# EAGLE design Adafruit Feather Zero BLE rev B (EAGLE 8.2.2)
COMPANY: ADAFRUIT INDUSTRIES; DRAWN: KTOWN; REV: B
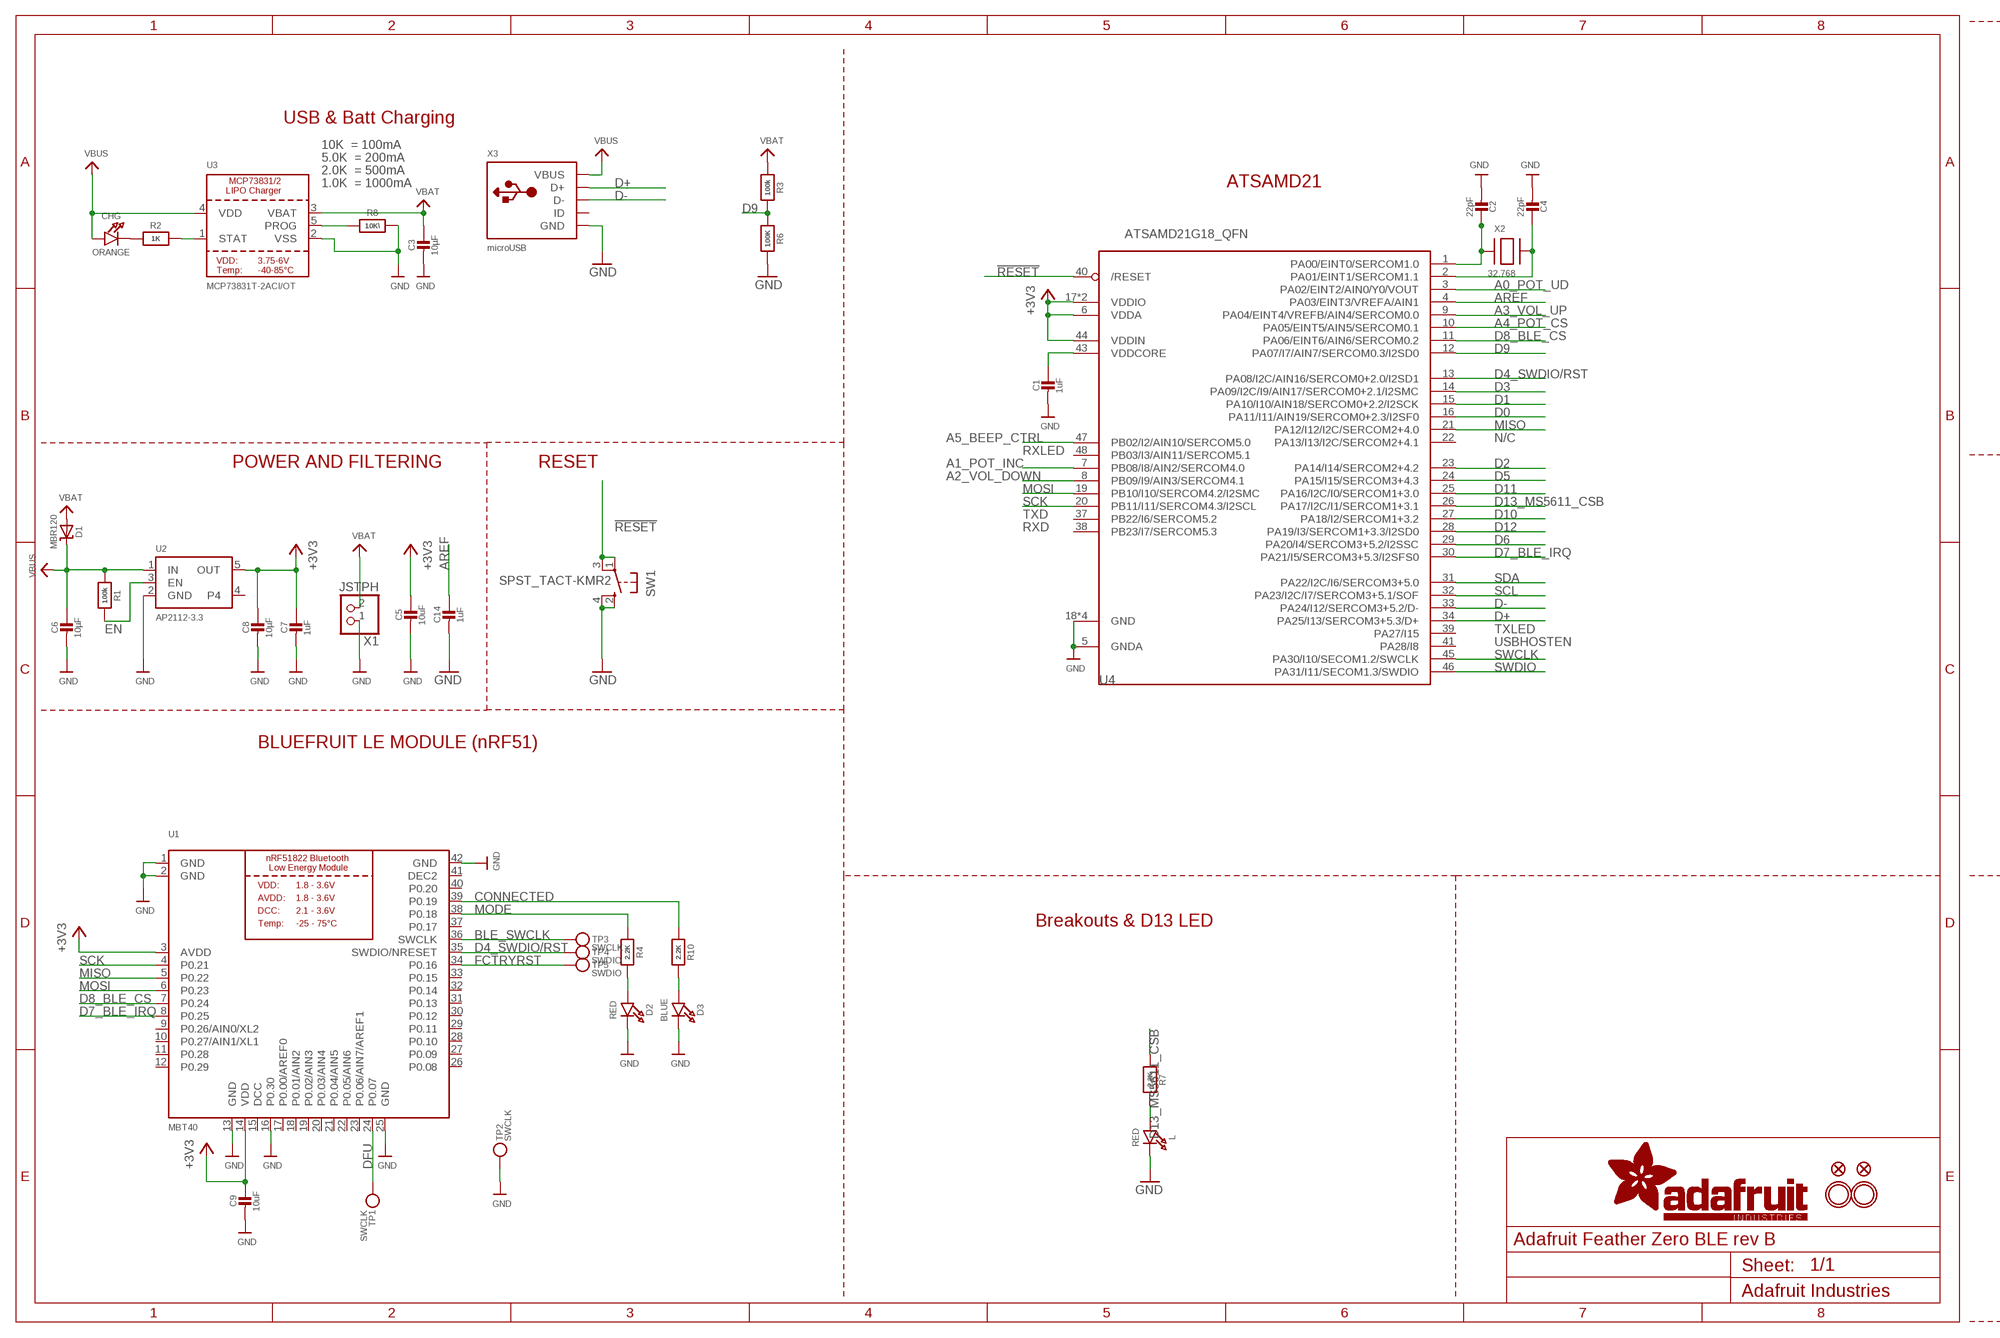
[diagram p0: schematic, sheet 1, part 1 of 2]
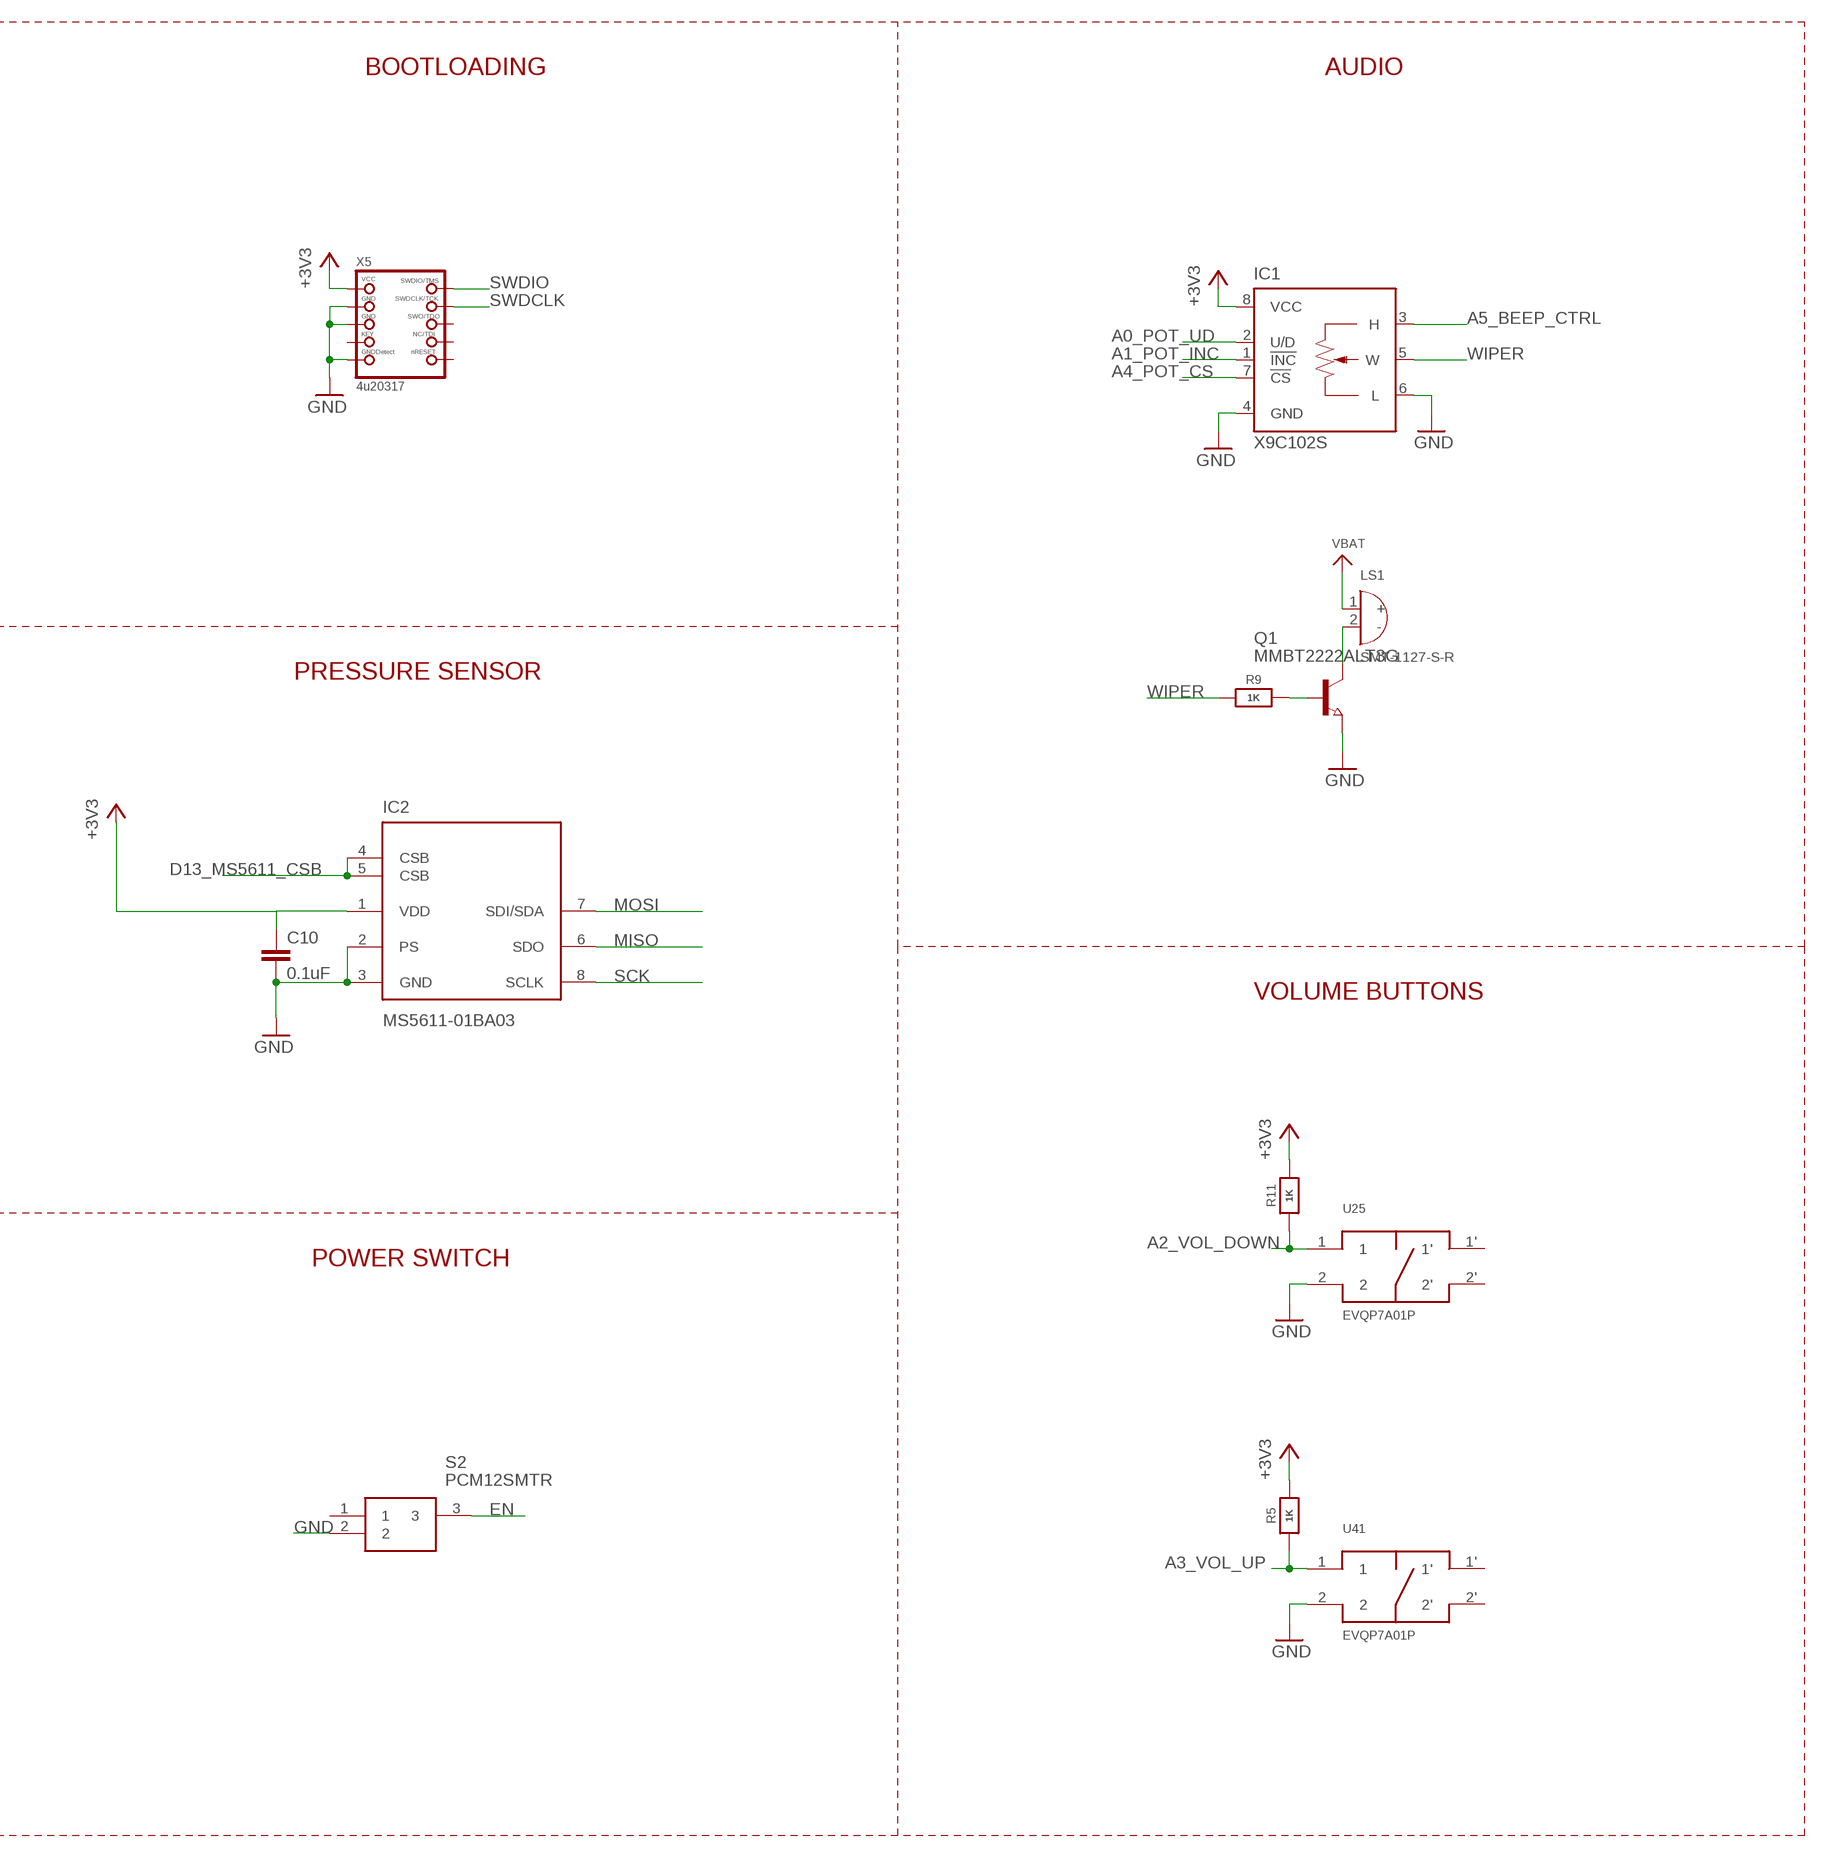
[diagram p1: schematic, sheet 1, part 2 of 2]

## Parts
C1  1uF  CAP_CERAMIC0603_NO  [0603-NO]
C2  22pF  CAP_CERAMIC0603_NO  [0603-NO]
C3  10µF  CAP_CERAMIC0805-NOOUTLINE  [0805-NO]
C4  22pF  CAP_CERAMIC0603_NO  [0603-NO]
C5  10uF  CAP_CERAMIC0805-NOOUTLINE  [0805-NO]
C6  10µF  CAP_CERAMIC0805-NOOUTLINE  [0805-NO]
C7  1uF  CAP_CERAMIC0603_NO  [0603-NO]
C8  10µF  CAP_CERAMIC0805-NOOUTLINE  [0805-NO]
C9  10uF  CAP_CERAMIC0805-NOOUTLINE  [0805-NO]
C10  0.1uF  C-EUC0805K  [C0805K]
C14  1uF  CAP_CERAMIC0603_NO  [0603-NO]
CHG  ORANGE  LED0805_NOOUTLINE  [CHIPLED_0805_NOOUTLINE]
D1  MBR120  DIODE-SCHOTTKYSOD-123  [SOD-123]
D2  RED  LED0805_NOOUTLINE  [CHIPLED_0805_NOOUTLINE]
D3  BLUE  LED0805_NOOUTLINE  [CHIPLED_0805_NOOUTLINE]
IC1  X9C102S  [SOIC08]
IC2  MS5611-01BA03  MS5611-01BA03UNO  [SON125P300X500X100-8N]
L  RED  LED0805_NOOUTLINE  [CHIPLED_0805_NOOUTLINE]
LS1  SMT-1127-S-R  [XDCR_SMT-1127-S-R]
Q1  MMBT2222ALT3G  NPN-TRANSISTOR_SOT23  [SOT23]
R1  100k  RESISTOR_0603_NOOUT  [0603-NO]
R2  1K  RESISTOR_0603_NOOUT  [0603-NO]
R3  100k  RESISTOR_0603_NOOUT  [0603-NO]
R4  2.2K  RESISTOR_0603_NOOUT  [0603-NO]
R5  1K  RESISTOR_0603_NOOUT  [0603-NO]
R6  100K  RESISTOR_0603_NOOUT  [0603-NO]
R7  2.2K  RESISTOR_0603_NOOUT  [0603-NO]
R8  10K\  RESISTOR_0603_NOOUT  [0603-NO]
R9  1K  RESISTOR_0603_NOOUT  [0603-NO]
R10  2.2K  RESISTOR_0603_NOOUT  [0603-NO]
R11  1K  RESISTOR_0603_NOOUT  [0603-NO]
S2  PCM12SMTR  [PCM12SMTR_1]
SW1  SPST_TACT-KMR2  [KMR2]
TP1  SWCLK  TESTPOINT1.5X2.0MM_NOCREAM  [PAD-1.5X2.0]
TP2  SWCLK  TESTPOINT1.5X2.0MM_NOCREAM  [PAD-1.5X2.0]
TP3  SWCLK  TESTPOINT1.5X2.0MM_NOCREAM  [PAD-1.5X2.0]
TP4  SWDIO  TESTPOINT1.5X2.0MM_NOCREAM  [PAD-1.5X2.0]
TP5  SWDIO  TESTPOINT1.5X2.0MM_NOCREAM  [PAD-1.5X2.0]
U1  MBT40  NRF51822_MODULE_MDBT40  [BLE_MODULE_RAYTAC_MDBT40]
U2  AP2112-3.3  VREG_SOT23-5  [SOT23-5]
U3  MCP73831T-2ACI/OT  MCP73831/2  [SOT23-5]
U4  ATSAMD21G18_QFN  ATSAMD21J_QFN  [TQFN48_7MM]
U25  EVQP7A01P  [EVQP7A01P]
U41  EVQP7A01P  [EVQP7A01P]
U$31  MOUNTINGHOLE2.5  [MOUNTINGHOLE_2.5_PLATED]
U$32  MOUNTINGHOLE2.5  [MOUNTINGHOLE_2.5_PLATED]
U$34  FIDUCIAL""  [FIDUCIAL_1MM]
U$35  FIDUCIAL""  [FIDUCIAL_1MM]
X1  JSTPH  CON_JST_PH_2PIN  [JSTPH2]
X2  32.768  XTAL-3.2X1.5  [XTAL3215]
X3  microUSB  USB_MICRO_20329_V2  [4UCONN_20329_V2]
X5  4u20317  JTAG-CORTEXBOXPOSTS  [2X05_1.27MM_BOX_POSTS]

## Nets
!RESET: SW1.1(P) SW1.3(P1) U4.40(/RESET)
+3V3: C5.1 C7.1 C8.1 C9.1 C10.1 IC1.8(VCC) IC2.1(VDD) R5.2 R11.2 U1.3(AVDD) U1.14(VDD) U2.5(OUT) U4.6(VDDA) U4.17(VDDIO) U4.36(VDDIO) U4.44(VDDIN) X5.1(VCC)
A0_POT_UD: IC1.2(U/D) U4.3(PA02/EINT2/AIN0/Y0/VOUT)
A1_POT_INC: IC1.1(!INC) U4.7(PB08/I8/AIN2/SERCOM4.0)
A2_VOL_DOWN: R11.1 U4.8(PB09/I9/AIN3/SERCOM4.1) U25.1
A3_VOL_UP: R5.1 U4.9(PA04/EINT4/VREFB/AIN4/SERCOM0.0) U41.1
A4_POT_CS: IC1.7(!CS) U4.10(PA05/EINT5/AIN5/SERCOM0.1)
A5_BEEP_CTRL: IC1.3(H) U4.47(PB02/I2/AIN10/SERCOM5.0)
AREF: C14.1 U4.4(PA03/EINT3/VREFA/AIN1)
BLE_SWCLK: TP3.P$1 U1.36(SWCLK)
CONNECTED: R10.1 U1.39(P0.19)
D0: U4.16(PA11/I11/AIN19/SERCOM0+2.3/I2SF0)
D1: U4.15(PA10/I10/AIN18/SERCOM0+2.2/I2SCK)
D2: U4.23(PA14/I14/SERCOM2+4.2)
D3: U4.14(PA09/I2C/I9/AIN17/SERCOM0+2.1/I2SMC)
D4_SWDIO/RST: TP4.P$1 U1.35(SWDIO/NRESET) U4.13(PA08/I2C/AIN16/SERCOM0+2.0/I2SD1)
D5: U4.24(PA15/I15/SERCOM3+4.3)
D6: U4.29(PA20/I4/SERCOM3+5.2/I2SSC)
D7_BLE_IRQ: U1.8(P0.25) U4.30(PA21/I5/SERCOM3+5.3/I2SFS0)
D8_BLE_CS: U1.7(P0.24) U4.11(PA06/EINT6/AIN6/SERCOM0.2)
D9: R3.2 R6.1 U4.12(PA07/I7/AIN7/SERCOM0.3/I2SD0)
D10: U4.27(PA18/I2/SERCOM1+3.2)
D11: U4.25(PA16/I2C/I0/SERCOM1+3.0)
D12: U4.28(PA19/I3/SERCOM1+3.3/I2SD0)
D13_MS5611_CSB: IC2.4(CSB) IC2.5(CSB) R7.1 U4.26(PA17/I2C/I1/SERCOM1+3.1)
D+: U4.34(PA25/I13/SERCOM3+5.3/D+) X3.D+
D-: U4.33(PA24/I12/SERCOM3+5.2/D-) X3.D-
DFU: TP1.P$1 U1.24(P0.07)
EN: R1.2 S2.3 U2.3(EN)
FCTRYRST: TP5.P$1 U1.34(P0.16)
GND: C1.2 C2.2 C3.2 C4.2 C5.2 C6.2 C7.2 C8.2 C9.2 C10.2 C14.2 D2.C D3.C IC1.4(GND) IC1.6(L) IC2.2(PS) IC2.3(GND) L.C Q1.2(E) R6.2 R8.2 S2.2 SW1.2(S) SW1.4(S1) TP2.P$1 U1.1(GND) U1.2(GND) U1.13(GND) U1.16(P0.30) U1.25(GND) U1.42(GND) U2.2(GND) U3.2(VSS) U4.5(GNDA) U4.18(GND) U4.35(GND) U4.42(GND) U4.THERMAL(GND) U25.2 U41.2 X1.1 X3.BASE@1(GND) X3.BASE@2(GND) X3.GND X3.SPRT@1(GND) X3.SPRT@2(GND) X3.SPRT@3(GND) X3.SPRT@4(GND) X5.3(GND) X5.5(GND) X5.9(GNDDETECT)
MISO: IC2.6(SDO) U1.5(P0.22) U4.21(PA12/I12/I2C/SERCOM2+4.0)
MODE: R4.1 U1.38(P0.18)
MOSI: IC2.7(SDI/SDA) U1.6(P0.23) U4.19(PB10/I10/SERCOM4.2/I2SMC)
N$1: CHG.C R2.1
N$2: L.A R7.2
N$3: R2.2 U3.1(STAT)
N$4: R8.1 U3.5(PROG)
N$5: C2.1 U4.1(PA00/EINT0/SERCOM1.0) X2.P$1
N$6: D2.A R4.2
N$7: C4.1 U4.2(PA01/EINT1/SERCOM1.1) X2.P$2
N$8: D3.A R10.2
N$9: Q1.1(B) R9.2
N$10: LS1.2(-) Q1.3(C)
SCK: IC2.8(SCLK) U1.4(P0.21) U4.20(PB11/I11/SERCOM4.3/I2SCL)
SCL: U4.32(PA23/I2C/I7/SERCOM3+5.1/SOF)
SDA: U4.31(PA22/I2C/I6/SERCOM3+5.0)
SWCLK: U4.45(PA30/I10/SECOM1.2/SWCLK)
SWDCLK: X5.4(SWDCLK)
SWDIO: U4.46(PA31/I11/SECOM1.3/SWDIO) X5.2(SWDIO)
VBAT: C3.1 D1.A LS1.1(+) R3.1 U3.3(VBAT) X1.2
VBUS: C6.1 CHG.A D1.C R1.1 U2.1(IN) U3.4(VDD) X3.VBUS
VDDCORE: C1.1 U4.43(VDDCORE)
WIPER: IC1.5(W) R9.1
Unconnected: S2.1 U1.9(P0.26/AIN0/XL2) U1.10(P0.27/AIN1/XL1) U1.11(P0.28) U1.12(P0.29) U1.17(P0.00/AREF0) U1.18(P0.01/AIN2) U1.19(P0.02/AIN3) U1.20(P0.03/AIN4) U1.21(P0.04/AIN5) U1.22(P0.05/AIN6) U1.23(P0.06/AIN7/AREF1) U1.26(P0.08) U1.27(P0.09) U1.28(P0.10) U1.29(P0.11) U1.30(P0.12) U1.31(P0.13) U1.32(P0.14) U1.33(P0.15) U1.37(P0.17) U1.40(P0.20) U2.4 U4.22(PA13/I13/I2C/SERCOM2+4.1) U4.37(PB22/I6/SERCOM5.2) U4.38(PB23/I7/SERCOM5.3) U4.39(PA27/I15) U4.41(PA28/I8) U4.48(PB03/I3/AIN11/SERCOM5.1) U25.1' U25.2' U41.1' U41.2' X3.ID X5.6(SWO) X5.7(KEY) X5.8(TDI) X5.10(NRESET)

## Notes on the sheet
- BOOTLOADING | AUDIO
- USB & Batt Charging
- 10K  = 100mA
- 5.0K  = 200mA
- 2.0K  = 500mA
- 1.0K  = 1000mA | ATSAMD21
- N/C
- RXLED
- POWER AND FILTERING | RESET
- PRESSURE SENSOR
- TXD
- RXD
- TXLED
- USBHOSTEN
- VOLUME BUTTONS
- BLUEFRUIT LE MODULE (nRF51)
- POWER SWITCH
- Breakouts & D13 LED

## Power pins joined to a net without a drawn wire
DCC: U1.15(DCC)
DEC2: U1.41(DEC2)

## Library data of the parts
C1-C9 C14 = microbuilder:CAP_CERAMIC: Ceramic Capacitors
C10 = rcl:C-EU: CAPACITOR, European symbol
CHG D2 D3 L = microbuilder:LED: LED
D1 = microbuilder:DIODE-SCHOTTKY
IC1 = pot-xicor:X9C102*: Digital POTENTIOMETER; MF: INTERSIL; MPN: X9C102SIZ; OC_FARNELL: 1562072; OC_NEWARK: 79K8947
IC2 = Measurement-Specialties:MS5611-01BA03: Variometer Module, with stainless steel cap
LS1 = SMT-1127-S-R:SMT-1127-S-R: Audio Indicator Transducer Electromagnetic 3.6Vpk 100mA Solder Pad 2.5Vpk 2231Hz to 3231Hz Surface Mount; AVAILABILITY: Good; DESCRIPTION: Black Passive Electromagnetic SMD Buzzer 3V 80mA 2700Hz 92dB 9x3.2mm; MF: PUI Audio; MP: BOT-03D-BUJEON, SMT-1127-S-R; PACKAGE: None; PRICE: 1.43 USD
Q1 = semicon-smd-ipc:NPN-TRANSISTOR_: NPN TRANSISTOR
R1-R11 = microbuilder:RESISTOR: Resistors
S2 = PCM12SMTR:PCM12SMTR: C & K COMPONENTS - PCM12SMTR - SWITCH, SPDT, 0.3A, 6VDC, SMD Source: Datasheet; ALLIED_NUMBER: 70417448; ALLIED_PRICE/STOCK: http://www.alliedelec.com/c-k-components-pcm12smtr/70417448/; DESCRIPTION: C & K COMPONENTS - PCM12SMTR - SWITCH, SPDT, 0.3A, 6VDC, SMD; HEIGHT: mm; MANUFACTURER_NAME: C & K COMPONENTS; MANUFACTURER_PART_NUMBER: PCM12SMTR; RS_PART_NUMBER: 7931721P; RS_PRICE/STOCK: http://uk.rs-online.com/web/p/products/7931721P
SW1 = adafruit:SPST_TACT: SMT 6mm switch, EVQQ2 series http://www.ladyada.net/library/eagle
TP1-TP5 = microbuilder:TESTPOINT: Test Point
U1 = microbuilder:NRF51822_MODULE_MDBT40: nRF51822 Bluetooth Low Energy Module
U2 = microbuilder:VREG_SOT23-5: SOT23-5 Fixed Voltage Regulators Part Current Out V Out V In V Dropout θJA (°C/W) TJ (°C) Digikey Part No. ADP121 150mA 3.3V 3.4-5.5V 0.09V @ 150mA -- -- ADP121-AUJZ33R7CT-ND ADP121 150mA 3.0V 3.1-5.5V 0.09V @ 150mA -- -- ADP121-AUJZ30R7CT-ND ADP122 300mA 3.3V 3.4-5.5V 0.085V @ 300mA -- --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
U3 = microbuilder:MCP73831/2: MCP73831/2 LIPO Charger VDD: 3.75 - 6V Temp -40 - 85°C Programmable Charge Rate: 15-500mA NOTE: STAT is a tri-state logic output on the MCP73831 and an open-drain output on the MCP73832. SOT23-5 with 4.2V output and tri-state logic on STAT = MCP73831T-2ACI/OT
U4 = microbuilder:ATSAMD21J
U25 U41 = EVQP7A01P:EVQP7A01P: EVQP7A01P Tactile Switch Surface Mount Right Angle
U$31 U$32 = microbuilder:MOUNTINGHOLE: Mounting Hole; BOM: EXCLUDE
U$34 U$35 = microbuilder:FIDUCIAL: Fiducial Alignment Points; BOM: EXCLUDE
X1 = microbuilder:CON_JST_PH_2PIN: JST 2-Pin Right-Angle Connector
X2 = adafruit2:XTAL: Low cost SMT crystals, no capacitors included
X3 = microbuilder:USB: USB Connectors USBMINIB - Surface Mount Female Mini-B USB Connector 4UConnector: 06564
X5 = microbuilder:JTAG-CORTEX: Serial Wire (SW-DP) Connector Standard 0.05" 10-pin connector is for use with the Cortex M and Cortex A SWD (serial wire debugger) interface (SW-DP) Connectors 2x05_1.27MM_SMT - Inexpensive surface-mount header with bare pins, compatible with standard 10-pin SWD cables (4UCON: 16846)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

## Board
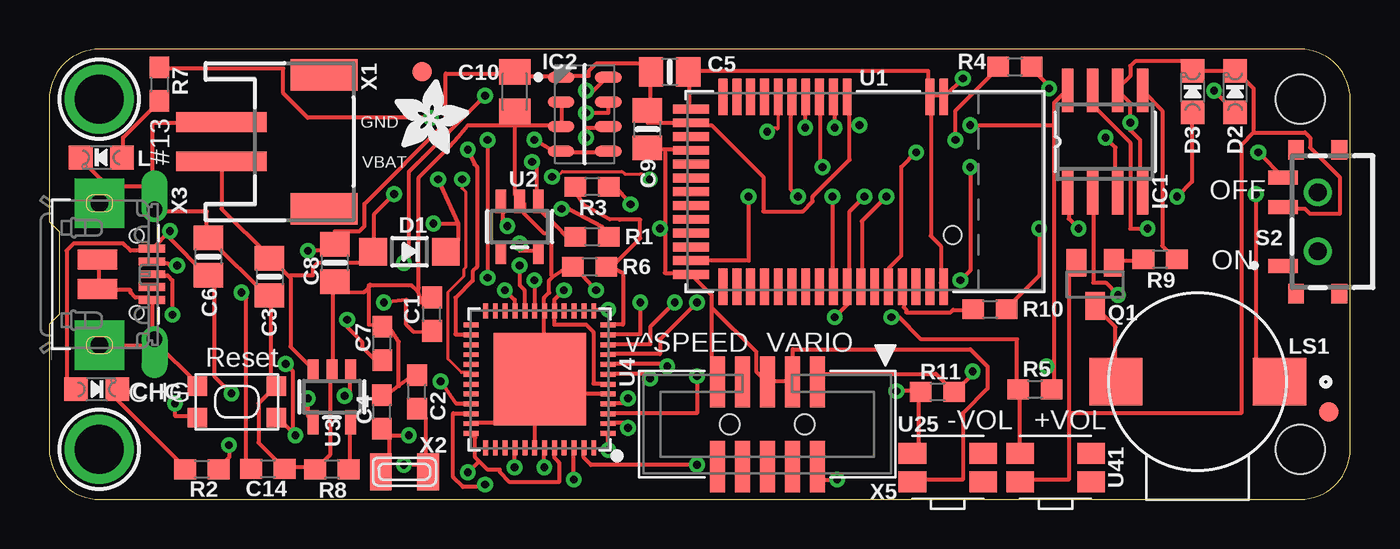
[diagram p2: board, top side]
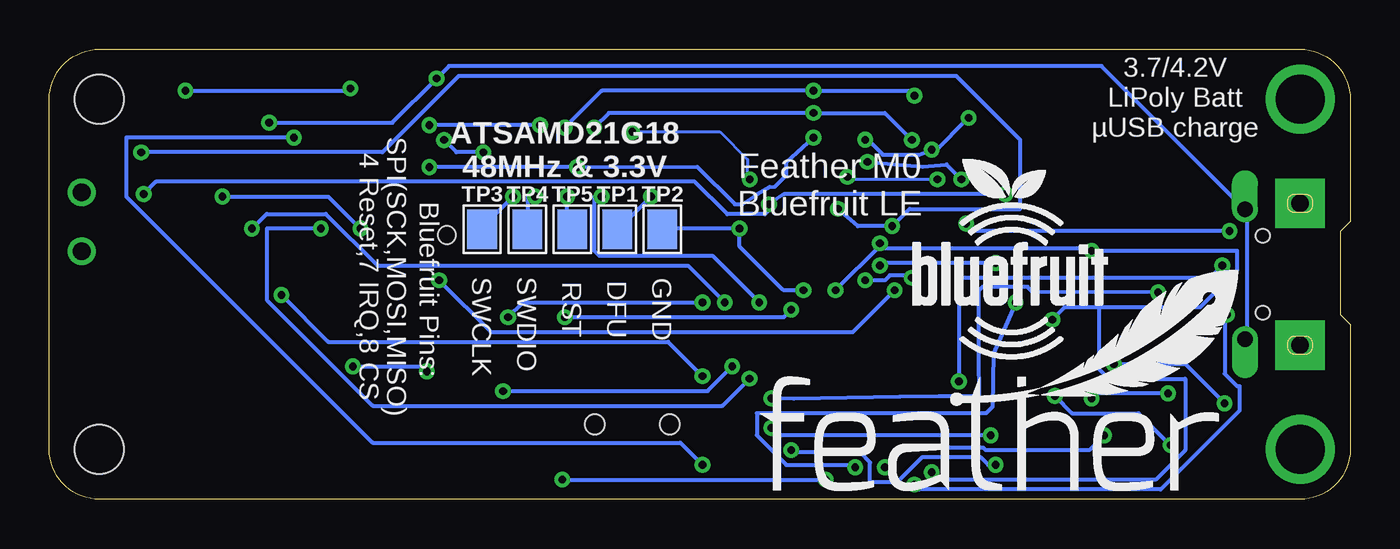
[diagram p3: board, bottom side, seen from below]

Size 66.04 x 22.86 mm. Coordinates in mm from the lower left corner, seen from the top.
Outline: 2.54,0 63.5,0 arc90 66.04,2.54 66.04,20.32 arc90 63.5,22.86 2.54,22.86 arc90 0,20.32 0,14.1 0.51,13.59 0.51,9.4 0,8.89 0,2.54 arc90 2.54,0
Copper layers (1*16): Top 0.035mm / dielectric 1.5mm / Bottom 0.035mm
Design rules "adafruit *": minimum track width 8mil, minimum drill 15.5mil, track to track 8mil, track to pad 8mil, pad to pad 8mil, via to via 8mil, smd to smd 8mil, copper to edge 10mil, drill to drill 8mil, minimum pad ring 10mil, minimum via ring 8mil, stop-mask expansion 2mil, vias tented up to drill 20mil, thermal gap 10mil
Holes 2.5 mm at 63.5,2.54 63.5,20.32

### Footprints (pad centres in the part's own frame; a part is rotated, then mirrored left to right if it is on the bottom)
0603-NO = smd 1.1 x 1: 1 -0.85,0; 2 0.85,0
0805-NO = smd 1.24 x 1.5: 1 -0.95,0; 2 0.95,0
C0805K = smd 1.3 x 1.6: 1 -1,0; 2 1,0
CHIPLED_0805_NOOUTLINE = smd 1.2 x 1.2: A 0,-1.05; C 0,1.05
SOD-123 = smd 1.4 x 1.4: A 1.85,0; C -1.85,0
SOIC08 = smd 0.6 x 2.2: 1 -1.905,-2.6; 2 -0.635,-2.6; 3 0.635,-2.6; 4 1.905,-2.6; 5 1.905,2.6; 6 0.635,2.6; 7 -0.635,2.6; 8 -1.905,2.6
SON125P300X500X100-8N = smd 1.35 x 0.55: 1 -1.2,1.875; 2 -1.2,0.625; 3 -1.2,-0.625; 4 -1.2,-1.875; 5 1.2,-1.875; 6 1.2,-0.625; 7 1.2,0.625; 8 1.2,1.875
XDCR_SMT-1127-S-R = smd 2.71 x 2.41: 1 -4.15,0; 2 4.15,0
SOT23 = smd 1 x 1.4: 1 -0.95,-1.1; 2 0.95,-1.1; 3 0,1.1
PCM12SMTR_1 = smd 0.7 x 1.5: 1 -2.25,1.75; 2 0.75,1.75; 3 2.25,1.75 | smd 1 x 0.8: 4 -3.65,1.1; 5 -3.65,-1.1; 6 3.65,1.1; 7 3.65,-1.1 | drill 0.9 pad 1.4: 8 -1.5,0; 9 1.5,0
KMR2 = smd 1 x 1: 1 2,0.8; 2 2,-0.8; 3 -2,0.8; 4 -2,-0.8
PAD-1.5X2.0 = smd 1.5 x 2: P$1 0,0
BLE_MODULE_RAYTAC_MDBT40 = smd 1.85 x 0.45: 1 -4.825,4; 2 -4.825,3.3; 3 -4.825,-0.9; 4 -4.825,-1.6; 5 -4.825,-2.3; 6 -4.825,-3; 7 -4.825,-3.7; 8 -4.825,-4.4; 9 -4.825,-5.1; 10 -4.825,-5.8; 11 -4.825,-6.5; 12 -4.825,-7.2; 26 4.825,-7.2; 27 4.825,-6.5; 28 4.825,-5.8; 29 4.825,-5.1; 30 4.825,-4.4; 31 4.825,-3.7; 32 4.825,-3; 33 4.825,-2.3; 34 4.825,-1.6; 35 4.825,-0.9; 36 4.825,-0.2; 37 4.825,0.5; 38 4.825,1.2; 39 4.825,1.9; 40 4.825,2.6; 41 4.825,3.3; 42 4.825,4 | smd 0.45 x 1.85: 13 -4.2,-8.825; 14 -3.5,-8.825; 15 -2.8,-8.825; 16 -2.1,-8.825; 17 -1.4,-8.825; 18 -0.7,-8.825; 19 0,-8.825; 20 0.7,-8.825; 21 1.4,-8.825; 22 2.1,-8.825; 23 2.8,-8.825; 24 3.5,-8.825; 25 4.2,-8.825 | hole 0.9: 2.2,4.45
SOT23-5 = smd 0.55 x 1.2: 1 -0.95,-1.3; 2 0,-1.3; 3 0.95,-1.3; 4 0.95,1.3; 5 -0.95,1.3
TQFN48_7MM = smd 0.25 x 0.75: 1 -2.75,-3.475; 2 -2.25,-3.475; 3 -1.75,-3.475; 4 -1.25,-3.475; 5 -0.75,-3.475; 6 -0.25,-3.475; 7 0.25,-3.475; 8 0.75,-3.475; 9 1.25,-3.475; 10 1.75,-3.475; 11 2.25,-3.475; 12 2.75,-3.475; 25 2.75,3.475; 26 2.25,3.475; 27 1.75,3.475; 28 1.25,3.475; 29 0.75,3.475; 30 0.25,3.475; 31 -0.25,3.475; 32 -0.75,3.475; 33 -1.25,3.475; 34 -1.75,3.475; 35 -2.25,3.475; 36 -2.75,3.475 | smd 0.75 x 0.25: 13 3.475,-2.75; 14 3.475,-2.25; 15 3.475,-1.75; 16 3.475,-1.25; 17 3.475,-0.75; 18 3.475,-0.25; 19 3.475,0.25; 20 3.475,0.75; 21 3.475,1.25; 22 3.475,1.75; 23 3.475,2.25; 24 3.475,2.75; 37 -3.475,2.75; 38 -3.475,2.25; 39 -3.475,1.75; 40 -3.475,1.25; 41 -3.475,0.75; 42 -3.475,0.25; 43 -3.475,-0.25; 44 -3.475,-0.75; 45 -3.475,-1.25; 46 -3.475,-1.75; 47 -3.475,-2.25; 48 -3.475,-2.75 | smd 4.7 x 4.7: THERMAL 0,0
EVQP7A01P = smd 1.4 x 1.05: 1 0,1.45; 1' 3.6,1.45; 2 0,0; 2' 3.6,0
MOUNTINGHOLE_2.5_PLATED = drill 2.5 pad 3.2: P$1 0,0
FIDUCIAL_1MM = smd 1 x 1: 1 0,0
JSTPH2 = smd 1 x 4.6: 1 -1,-3.7; 2 1,-3.7 | smd 1.6 x 3.4: NC1 -3.4,1.5; NC2 3.4,1.5
XTAL3215 = smd 1.1 x 1.9: P$1 1.2,0; P$2 -1.2,0
4UCONN_20329_V2 = smd 1 x 2: BASE@1 -0.75,-2; BASE@2 0.75,-2 | smd 0.4 x 1.35: D+ 0,0.775; D- -0.65,0.775; GND 1.3,0.775; ID 0.65,0.775; VBUS -1.3,0.775 | drill 0.8 pad 1.2 offset: SPRT@1 -3.3,0.9; SPRT@2 3.3,0.9 | drill 0.9 pad 2.5 square: SPRT@3 -3.6,-1.9; SPRT@4 3.6,-1.9 | hole 0.7: -1.95,0; 1.95,0
2X05_1.27MM_BOX_POSTS = smd 0.76 x 2.6: 1 -2.54,-2.15; 2 -2.54,2.15; 3 -1.27,-2.15; 4 -1.27,2.15; 5 0,-2.15; 6 0,2.15; 7 1.27,-2.15; 8 1.27,2.15; 9 2.54,-2.15; 10 2.54,2.15 | hole 1: -1.905,0; 1.905,0

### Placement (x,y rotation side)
C1  19.43,9.4 90 top
C2  18.67,5.46 90 top
C3  11.18,11.3 270 top
C4  16.89,4.45 90 top
C5  31.5,21.72 0 top
C6  8.09,12.32 90 top
C7  16.91,7.92 90 top
C8  14.49,12.01 270 top
C9  30.35,18.8 270 top
C10  23.62,20.7 270 top
C14  11.1,1.55 0 top
CHG  2.41,5.59 270 top
D1  18.29,12.57 180 top
D2  60.2,20.7 0 top
D3  58.04,20.7 0 top
IC1  53.59,18.16 0 top
IC2  27.18,19.56 0 top
L  2.65,17.36 90 top
LS1  58.29,5.97 180 top
Q1  53.09,10.92 180 top
R1  27.56,13.34 0 top
R2  7.75,1.52 0 top
R3  27.56,15.88 180 top
R4  49.02,21.97 0 top
R5  50.04,5.59 0 top
R6  27.43,11.81 180 top
R7  5.59,21.08 270 top
R8  14.35,1.52 180 top
R9  56.39,12.19 180 top
R10  47.75,9.65 0 top
R11  45.09,5.46 0 top
S2  64.39,14.1 90 top
SW1  9.53,4.95 180 top
TP1  37.21,13.72 0 bottom
TP2  34.92,13.72 0 bottom
TP3  44.07,13.72 0 bottom
TP4  41.78,13.72 0 bottom
TP5  39.5,13.72 0 bottom
U1  41.4,15.62 270 top
U2  23.88,13.84 180 top
U3  14.35,5.21 180 top
U4  24.89,6.1 90 top
U25  43.81,0.89 0 top
U41  49.28,0.89 0 top
U$7  [ADAFRUIT_3.5MM]  17.53,17.53 0 top
U$9  [FEATHERLOGO]  29.97,0.38 0 bottom
U$26  [BLUEFRUITLOGO_100MM]  22.23,7.11 0 bottom
U$31  2.54,20.32 270 top
U$32  2.54,2.54 270 top
U$34  18.92,21.72 270 top
U$35  64.94,4.45 270 top
X1  12.45,18.16 270 top
X2  18.03,1.4 0 top
X3  4.45,11.43 270 top
X5  36.45,3.81 180 top

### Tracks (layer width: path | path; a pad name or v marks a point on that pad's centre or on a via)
!RESET  (via drill 0.39)
  Top 0.203: v23.62,1.62 23.62,2.5 U4.40 | SW1.3 11.62,4.12 v12.5,3.25 12.38,3.5 12.38,6.5 v12,6.88 | v6.38,4.88 6.38,4.25 7.5,4.25 SW1.1
  Bottom 0.203: v23.62,1.62 22.62,2.62 18.62,2.62 18.5,2.5 13.25,2.5 v12.5,3.25 | v6.38,4.88 8.38,6.88 v12,6.88
+3V3  (via drill 0.39)
  Top 0.203: X5.1 39,6 39,6.38 45,6.38 45.88,5.5 R11.2 46,5.5 46.88,6.38 v46.88,6.5 | 51,19 51,20.12 51.62,20.75 IC1.8 | 51,19 51,6.75 | 51,6.75 51,5.62 R5.2 | 51,6.75 v50.62,6.75 | 40.62,19 40.62,17.25 38.75,15.38 38.75,15.12 38.25,14.62 36.25,14.62 36.25,16.38 33.62,19 32.62,19 U1.14 32.5,19.12 30.38,19.12 30.38,19.62 C9.1 30.38,19.75 30.5,19.88 30.5,21.62 C5.1 30.5,21.75 30.5,22.12 27.75,22.12 27.38,21.75 27.38,21.5 26,21.5 IC2.1 25.88,21.5 23.62,21.5 23.62,21.62 C10.1 23.5,21.62 20.12,21.62 20.12,19.12 16,15 16,13.88 15.75,13.62 14.5,13.62 14.5,13 C8.1 14.38,12.88 14.38,12.62 v13.12,12.62 | 40.62,19 40.62,20.38 U1.3 | U4.6 28.25,5.88 27.62,5.88 27.62,8.5 27.25,8.88 25.62,8.88 25.62,9.5 U4.17 25.62,9.62 25.62,10.12 v26.12,10.62 | 21.81,1.94 22.25,1.5 22.88,1.5 22.88,1.38 23.38,0.88 25.88,0.88 25.88,1.88 25.62,2.12 25.62,2.5 U4.44 | 21.81,1.94 21.62,2.12 21.62,3.12 21.5,3.25 U4.36 | v15.12,9.12 15.12,8.75 15.88,8 15.88,7.75 16.51,7.11 17.12,7.12 C7.1 | v23.88,13 23.88,12.62 24.75,12.62 U2.5 | v21.25,1.38 21.81,1.94 | v46.75,19 51,19 | 40.62,19 v41.12,19
  Bottom 0.203: v46.88,6.5 47.12,6.75 v50.62,6.75 | v15.12,9.12 14.5,9.75 12.75,9.75 | 12.75,9.75 7.62,9.75 5.75,11.62 5.75,12.62 v13.12,12.62 13.25,12.75 23.62,12.75 v23.88,13 23.88,12.88 v26.12,10.62 | v21.25,1.38 20.88,1 9.88,1 8.38,2.5 8.38,6.12 12.25,6.12 12.75,6.62 12.75,9.75 | v41.12,19 v46.75,19
A0_POT_UD  (via drill 0.39)
  Top 0.203: v32.88,6.25 32.88,4.38 28.38,4.38 U4.3 | v54.25,10.38 53.62,11 53,11 53,15.5 IC1.2
  Bottom 0.203: v32.88,6.25 34.62,8 51.88,8 v54.25,10.38
A1_POT_INC  (via drill 0.39)
  Top 0.203: v30.5,6.12 30.5,6.38 28.38,6.38 U4.7 | v52.25,13.75 51.75,14.25 51.75,15.5 IC1.1
  Bottom 0.203: v30.5,6.12 31.88,4.75 49.62,4.75 55,10.12 55,13.75 v52.25,13.75
A2_VOL_DOWN  (via drill 0.39)
  Top 0.203: v31.38,6.75 31.38,6.88 28.38,6.88 U4.8 | v43,5.5 44.12,5.5 R11.1 44.12,5.38 44.12,2.62 43.88,2.38 U25.1
  Bottom 0.203: v31.38,6.75 32.62,5.5 v43,5.5
A3_VOL_UP  (via drill 0.39)
  Top 0.203: v32.88,10 31,8.12 31,7.38 28.38,7.38 U4.9 | v42.75,9.25 43.12,9.25 44.25,8.12 49.12,8.12 49.12,5.62 R5.1 49.25,5.5 49.25,2.38 U41.1
  Bottom 0.203: v32.88,10 42,10 v42.75,9.25
A4_POT_CS  (via drill 0.39)
  Top 0.203: v31.75,10 30.5,8.75 30.5,7.88 28.38,7.88 U4.10 | v55.75,13.75 54.88,13.75 54.88,18.12 53,20 53,20.75 IC1.7
  Bottom 0.203: v31.75,10 33.62,11.88 49.38,11.88 52,14.5 55,14.5 v55.75,13.75
A5_BEEP_CTRL  (via drill 0.39)
  Top 0.203: v32.88,1.75 27.5,1.75 27.12,2.12 27.12,2.5 U4.47 | v53.62,18.38 54.12,17.88 54.12,15.62 IC1.3
  Bottom 0.203: v32.88,1.75 34,2.88 49.62,2.88 62.12,15.38 62.12,18.38 v53.62,18.38
AREF  (via drill 0.39)
  Top 0.203: v29.38,5.12 29.38,4.88 28.38,4.88 U4.4 | v9.75,10.5 10,10.25 10,1.75 10.12,1.62 C14.1
  Bottom 0.203: v29.38,5.12 28.25,5.11 22.86,5.21 20.86,5.24 18.86,5.24 18.88,7.25 18.88,10.59 18.67,10.79 16.38,10.79 16.13,10.54 v9.75,10.5
BLE_SWCLK  (via drill 0.39)
  Top 0.203: v42.5,15.38 41.25,14.12 41.25,10.88 U1.36
  Bottom 0.203: v42.5,15.38 44.12,13.75 TP3.P$1
CONNECTED
  Top 0.203: R10.1 46.88,9.62 45.88,9.62 45.75,9.5 43.5,9.5 43.5,9.62 43.38,9.75 43.38,10.75 U1.39
D4_SWDIO/RST  (via drill 0.39)
  Top 0.203: v28.38,9.62 27.75,9.62 U4.13 | v39.88,9.25 40.5,9.88 40.5,10.75 U1.35 40.62,10.88 40.62,14.62 v41.38,15.38
  Bottom 0.203: v28.38,9.62 28.75,9.25 v39.88,9.25 | v41.38,15.38 41.75,15.38 41.75,13.75 TP4.P$1
D7_BLE_IRQ  (via drill 0.39)
  Top 0.152: U4.30 21.32,6.44 20.93,6.44 20.24,7.12 20.24,10.52 21.05,11.33 21.05,11.69 21.13,11.77 21.13,15.62 20.95,15.8 v20.95,16.26 | U1.8 37,18.84 | 37,18.84 36.96,18.8 | 37,18.84 36.62,18.84 v36.45,18.67 | v25.53,16.38 25.77,16.38 26.04,16.65 29.07,16.65 29.22,16.51 29.97,16.51 30.1,16.51 30.35,16.26 v30.48,16.26
  Bottom 0.152: v36.45,18.67 32,18.67 30.59,17.26 30.59,16.91 30.61,16.64 30.48,16.51 v30.48,16.26 | v20.95,16.26 25.4,16.26 v25.53,16.38
D8_BLE_CS  (via drill 0.39)
  Top 0.203: v30,10 30,8.38 28.38,8.38 U4.11 | v38,15.38 37.62,15.75 37.62,20.38 U1.7
  Bottom 0.203: v30,10 32.38,12.38 38.12,12.38 38.38,12.62 38.38,15.38 v38,15.38
D9
  Top 0.203: U4.12 28.38,8.88 29.12,8.88 29.12,11.5 28.38,11.87 R6.1 28.75,12 30,13.25 30,14.21 28.97,14.21 28.45,14.22 27.12,14.97 26.38,16.12 R3.2
D13_MS5611_CSB  (via drill 0.39)
  Top 0.203: v21.25,17.76 21.59,17.02 21.72,16.89 21.72,11.81 21.5,11.59 21.5,11.11 20.62,10.24 20.62,8.38 21.38,8.38 U4.26 | v24.62,18.26 25.88,17.5 25.88,17.62 IC2.4 26,17.62 28.38,17.62 IC2.5 | v19.38,19.38 13.12,19.38 11.88,20.62 11.88,21.88 5.62,21.88 R7.1
  Bottom 0.203: v24.62,18.26 24.38,18.16 23.72,17.5 21.88,17.5 v21.25,17.76 21.12,17.63 v19.38,19.38
D+  (via drill 0.39)
  Top 0.203: v22.12,0.75 22.12,0.62 21,0.62 20.5,1.12 20.5,4.38 21.38,4.38 U4.34 | v6.25,9.38 6.25,11.12 6,11.38 5.25,11.38 X3.D+
  Bottom 0.203: v22.12,0.75 21.88,0.5 9.62,0.5 5.62,4.5 5.62,5.75 5.75,5.75 6.38,6.38 6.38,9.38 v6.25,9.38
D-  (via drill 0.39)
  Top 0.203: v19.87,5.99 20.63,4.88 21.38,4.88 U4.33 | v6.5,11.88 6.12,11.88 6,12 5.25,12 X3.D-
  Bottom 0.203: v19.87,5.99 19.87,11.25 7.12,11.25 v6.5,11.88
DFU  (via drill 0.39)
  Top 0.203: v35.5,15.38 35.5,12.12 32.62,12.12 U1.24
  Bottom 0.203: v35.5,15.38 37.12,13.75 TP1.P$1
EN  (via drill 0.39)
  Top 0.203: v26,14.75 26.4,14.75 28.07,13.84 28.12,13.61 28.11,13.37 R1.2 | v23.25,13.88 23,14.12 23,15.12 U2.3 | v61.38,17.62 62.62,16.38 S2.3
  Bottom 0.203: v26,14.75 25,13.88 v23.25,13.88 22.38,14.75 16.75,14.75 16.75,18.25 20,21.5 45.25,21.5 49.12,17.62 v61.38,17.62
FCTRYRST  (via drill 0.39)
  Top 0.203: v39.75,15.38 39.75,10.88 U1.34
  Bottom 0.203: v39.75,15.38 39.75,13.75 39.5,13.75 TP5.P$1
GND  (via drill 0.39)
  Top 0.152: X3.SPRT@3 2.54,15.53 2.94,15.93 | 5.25,8.25 4.83,7.83 X3.SPRT@4
  Top 0.203: U1.13 32.5,19.88 32.5,21.62 C5.2 32.5,21.75 44.62,21.75 44.62,20.5 U1.2 | U1.2 44.75,20.5 45.38,20.5 U1.1 45.5,20.5 v46.38,21.38 | U1.42 45.38,10.88 45.25,11 45.25,12.88 44.75,13.38 44.75,20.38 U1.2 | 51.75,4.38 51.75,11.62 52.12,12 Q1.2 | 51.75,4.38 51.75,1 49.38,1 U41.2 | IC1.4 55.38,15.62 55.38,18.25 54.88,18.75 v54.88,19.12 54.88,20.12 54.25,20.75 IC1.6 54.25,20.88 54.88,21.5 54.88,22 55.12,22.25 58,22.25 58,21.88 D3.C 58.12,21.75 60.12,21.75 D2.C 60.25,21.75 61.12,20.88 61.12,18.62 | 61.12,18.62 63.75,18.62 64,18.38 64,17.88 65.5,16.38 65.5,14.5 64,14.5 63.75,14.75 62.75,14.75 S2.2 | 51.75,4.38 60.5,4.38 60.5,18 61.12,18.62 | U25.2 43.88,1 46.38,1 46.38,4.38 47.62,5.62 47.62,6.75 46.75,7.62 37.75,7.62 37.75,6 X5.3 37.62,6 36.5,6 X5.5 36.38,6 35.88,6.5 35.88,7.5 33.62,9.75 | 31.25,17.75 32.5,17.75 U1.16 | 31.25,17.75 30.38,17.75 C9.2 | 31.25,17.75 31.25,13.75 | 31.25,13.75 31.25,11.5 32.5,11.5 U1.25 32.62,11.38 33.62,10.38 33.62,9.75 | 31.25,13.75 v31,13.75 | 33.62,9.75 33.62,6.25 33.88,6 X5.9 | IC2.2 26,20.12 26,19 IC2.3 25.88,19 23.62,19 | 23.62,19 23.62,19.62 C10.2 | 23.62,19 23.62,15.5 23.88,15.25 U2.2 24,15.12 24.12,15 24.12,14.5 25.12,13.5 25.5,13.5 25.5,11.38 25.56,11.31 | 24.62,3.88 24.62,5.75 24.88,6 U4.THERMAL | 24.62,3.88 24.62,2.62 U4.42 | 24.62,3.88 21.5,3.88 U4.35 | 24.62,3.88 U4.THERMAL | 25.12,5.38 24.88,5.38 U4.THERMAL | 25.12,5.38 28.25,5.38 U4.5 | 25.12,5.38 25.12,9.5 U4.18 25.12,9.62 25.12,10.25 25.38,10.5 25.38,11.12 25.56,11.31 | 25.12,5.38 U4.THERMAL | 25.56,11.31 26.37,11.87 R6.2 26.62,11.87 v27.75,10.62 | 17.75,5.76 18.61,6.39 18.61,6.38 C2.2
  Top 0.203: 17.75,5.76 17.25,5.38 C4.2 | 17.75,5.76 17.75,8 17.25,8.75 C7.2 16.23,8.88 16.23,10.88 16.34,10.88 | 18.69,10.57 18.38,10.88 16.34,10.88 | 18.69,10.57 18.88,10 19,10 19.5,10.39 C1.2 | 14.38,10.5 14.38,11 C8.2 14.38,10.5 | 14.38,10.5 14.38,6.62 U3.2 14.25,6.5 14.25,2.25 13.62,1.62 R8.2 13.5,1.62 12,1.62 C14.2 11.88,1.62 10.62,2.88 10.62,4.88 11.5,5.75 SW1.4 11.5,5.88 11.25,6.12 11.25,10.25 C3.2 11.12,10.25 8.12,13.25 C6.2 8,13.38 8,14.62 5.38,14.62 X3.SPRT@1 | 14.38,10.5 16,10.54 16.34,10.88 | X3.BASE@1 2.5,12.12 2.5,10.75 X3.BASE@2 2.5,10.62 4.12,10.62 4.12,10.5 4.38,10.25 5.12,10.25 X3.GND 5.25,10.12 5.25,8.25 X3.SPRT@2 5.38,8.12 5.38,8 7.5,5.88 SW1.2 | 5.25,15.88 3,15.88 2.94,15.93 1.62,17.25 L.C | 5.25,15.88 5.25,14.75 X3.SPRT@1 | 5.25,15.88 5.25,19.12 8.62,19.12 X1.1 | 5.25,15.88 X3.SPRT@1 | 23.62,19 21.25,19 20.74,18.38 20.32,17.91 18.75,16.34 18.75,10.76 18.69,10.57
  Bottom 0.203: v54.88,19.12 48.62,19.12 v46.38,21.38 45.75,22 12.62,22 5.38,14.75 X3.SPRT@1 5.25,14.62 5.25,8.25 X3.SPRT@2 | TP2.P$1 34.88,13.75 v31,13.75 31,12.84 28.83,10.67 28.76,10.62 v27.75,10.62
MISO  (via drill 0.39)
  Top 0.203: v23.12,10.62 23.62,10.12 23.62,9.62 U4.21 | v46.25,11.12 46.75,11.62 v46.75,16.88 | v39.25,16.88 39.12,17 39.12,20.38 U1.5 | v27.25,18.38 27.25,18.88 28.38,18.88 IC2.6
  Bottom 0.203: v23.12,10.62 25.25,8.5 43.62,8.5 v46.25,11.12 | v46.75,16.88 v39.25,16.88 33.15,16.89 31.24,14.99 30.86,14.99 30.1,15.49 29.48,15.86 29.21,15.88 28.62,16.46 28.62,17.13 v27.25,18.38
MODE  (via drill 0.39)
  Top 0.203: v46,18.25 46,19.75 48.12,21.88 R4.1 | v44,17.62 43.25,16.88 43.25,12.38 42.62,11.75 42.62,10.88 U1.38
  Bottom 0.203: v46,18.25 45.38,17.62 v44,17.62
MOSI  (via drill 0.39)
  Top 0.203: v24.62,11.12 24.62,9.62 U4.19 | v22.25,18.25 v22.25,11.25 | v27.25,19.62 28.38,19.62 28.38,20.12 IC2.7 | v38.38,18.88 38.38,20.38 U1.6
  Bottom 0.203: v24.62,11.12 23.62,11.12 23.38,11.38 22.38,11.38 v22.25,11.25 | v22.25,18.25 23.62,19.62 v27.25,19.62 37.62,19.62 v38.38,18.88
N$1
  Top 0.203: R2.1 6.88,1.62 3.5,5 3.5,5.5 CHG.C
N$2
  Top 0.203: R7.2 5.5,20.12 3.75,18.38 3.75,17.38 L.A
N$3  (via drill 0.39)
  Top 0.203: v9.12,2.75 9.12,2.12 8.62,1.62 R2.2 | v15,5.25 15.25,5.5 15.25,6.5 U3.1
  Bottom 0.203: v9.12,2.75 10.75,4.38 14.12,4.38 v15,5.25
N$4
  Top 0.203: R8.1 15.25,1.62 15.25,3.88 U3.5
N$5  (via drill 0.39)
  Top 0.203: v28.38,2.5 28.38,3.25 U4.1 | 19.12,1.75 v18,1.75 | 19.12,1.75 19.12,1.5 X2.P$1 19.12,1.75 | 19.12,1.75 19.12,3.88 19.12,4.13 C2.1
  Bottom 0.203: v28.38,2.5 28.25,2.38 24.88,2.38 24.38,1.88 24.38,0.88 23,0.88 21.75,2.12 18.75,2.12 18.38,1.75 v18,1.75
N$6  (via drill 0.39)
  Top 0.203: v50.75,20.88 50.75,21 49.88,21.88 R4.2 | v59.12,20.75 60.12,19.75 D2.A
  Bottom 0.203: v50.75,20.88 50.88,20.75 v59.12,20.75
N$7  (via drill 0.39)
  Top 0.203: v29.38,3.62 29.38,3.88 28.38,3.88 U4.2 | 17.25,3.25 v18.25,3.25 | 17.25,3.25 17.25,3.5 C4.1 17.25,3.25 | 17.25,3.25 17.25,1.88 16.88,1.5 X2.P$2
  Bottom 0.203: v29.38,3.62 29,3.25 v18.25,3.25
N$8  (via drill 0.39)
  Top 0.203: v50.25,13.75 50.25,11.38 48.62,9.75 R10.2 | v57.25,15.38 58,16.12 58,19.62 D3.A
  Bottom 0.203: v50.25,13.75 51.88,15.38 v57.25,15.38
N$9
  Top 0.203: R9.2 55.5,12.12 54.12,12.12 Q1.1
N$10
  Top 0.203: Q1.3 53.12,9.75 54.12,8.75 54.12,6 LS1.2
SCK  (via drill 0.39)
  Top 0.203: v23.88,11.88 23.88,10.88 24.12,10.62 24.12,9.62 U4.20 | v18,12 18.25,12.25 18.25,16.62 v22.12,20.5 | v27.25,20.75 27.62,20.75 28.38,21.5 IC2.8 | v39.88,18.88 39.88,20.38 U1.4
  Bottom 0.203: v23.88,11.88 23.75,12 v18,12 | v22.12,20.5 22.38,20.75 v27.25,20.75 38,20.75 v39.88,18.88
SWDIO  (via drill 0.39)
  Top 0.203: v26.62,1 26.62,2.5 U4.46 | v40,1 39,1 39,1.62 X5.2
  Bottom 0.203: v40,1 v26.62,1
VBAT  (via drill 0.39)
  Top 0.203: 12.19,11.31 11.25,12.25 C3.1 11.12,12.38 8.75,14.75 8.75,17.12 X1.2 | 12.19,11.31 12.25,11.25 12.25,7.75 13.38,6.62 U3.3 | v29.5,14.98 28.51,16.13 R3.1 | v17.5,15.5 16.5,14.5 16.5,12.62 D1.A 16.38,12.5 16.38,12 13.62,12 13.38,11.75 13.38,11.38 12.25,11.38 12.19,11.31 | v61.25,15.5 61.25,7.12 62.38,6 LS1.1
  Bottom 0.203: v17.5,15.5 28.75,15.5 v29.5,14.98 29.5,14.86 29.5,14.69 29.72,14.48 31.62,14.48 33.27,16.13 60.62,16.12 v61.25,15.5
VBUS  (via drill 0.39)
  Top 0.203: v13.12,5.12 13.12,4.25 13.38,4 U3.4 | v9.25,5.38 8.38,6.25 8.38,11 8.12,11.25 C6.1 8,11.38 6,13.38 v6.12,13.62 5.25,12.75 X3.VBUS 5.12,12.62 4.12,12.62 3.75,13 1.25,13 0.88,12.62 0.88,6 1.25,5.62 CHG.A | R1.1 26.23,13.37 25.75,13.88 24.88,14.75 24.88,15.12 U2.1 24.75,15.25 24.75,17 24.77,17.02 v24.5,17.14 | v19.73,16.25 20.75,14 | 20.75,14 20.75,13.12 20.25,12.62 D1.C | v19.5,14 20.75,14
  Bottom 0.203: v13.12,5.12 12.88,5.38 v9.25,5.38 | v19.73,16.25 20.49,17.01 21.72,16.89 24.38,17.14 v24.5,17.14 | v19.5,14 19.12,13.62 v6.12,13.62
VDDCORE  (via drill 0.39)
  Top 0.203: v25.12,1.62 25.12,2.5 U4.43 | v16.98,10 18.12,10.13 18.12,8.88 18.49,8.51 C1.1
  Bottom 0.203: v25.12,1.62 25.25,1.75 28.62,1.75 30.12,3.25 30.12,4.38 18.48,4.38 18.16,4.7 18.12,7.38 v16.98,10
WIPER
  Top 0.203: R9.1 57.12,12.25 56.5,12.88 56.5,19.75 IC1.5

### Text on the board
tPlace: GND | #13 | VBAT | OFF | ON | v^SPEED | VARIO | Reset | CHG | -VOL | +VOL
bPlace: 3.7/4.2V / LiPoly Batt / µUSB charge | ATSAMD21G18 / 48MHz & 3.3V | Feather M0 / Bluefruit LE | Bluefruit Pins: | SPI(SCK,MOSI,MISO) | 4 Reset,7 IRQ,8 CS | GND | DFU | RST | SWDIO | SWCLK

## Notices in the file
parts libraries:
microbuilder: This work is placed in the public domain, and may be freely used for commercial and non-commercial work with the following conditions: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
